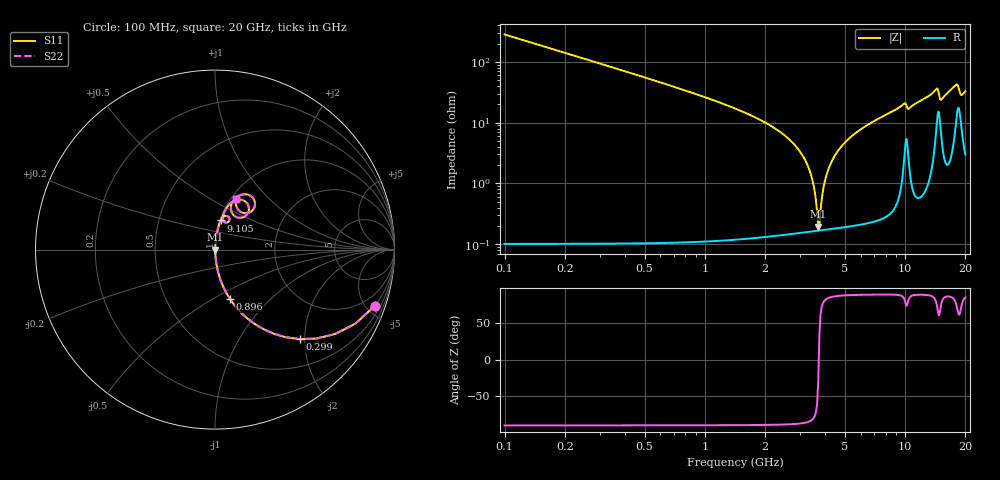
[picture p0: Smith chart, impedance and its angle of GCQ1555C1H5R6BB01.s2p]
!Murata Part Number: GCQ1555C1H5R6BB01
!These Parameters are Measured in Series Mode Connection
!Data Generated on Jan 08, 2026
!  o--ll--o
!Port1  Port2
!  o------o
!Operation Temp=25[degC], DC Bias Voltage=0[V]
!Freq. Start=100[MHz] Stop=20[GHz] 401[Steps]
# Hz S RI R 50
!Freq.(Hz) S11(Real) S11(Imag) S21(Real) S21(Imag) S12(Real) S12(Imag) S22(Real) S22(Imag)
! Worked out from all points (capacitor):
!   401 points, 100 MHz to 20 GHz, reference 50 ohm
!   read as one part in series: C = 5.6 pF near 199.5 MHz
!   lowest |Z| = 194 mohm at 3.682 GHz (marker M1)
!   series resonance near 3.706 GHz, so ESL is about 330 pH
!   S11 on the Smith chart (normalised r, x): 100 MHz: 1.00, -5.68; 299 MHz: 1.00, -1.89; 896 MHz: 1.00, -0.60; 9.105 GHz: 1.01, +0.34; 20 GHz: 1.06, +0.66
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1e8  0.8896 -0.3132  0.1104 0.3132  0.1104 0.3132  0.8896 -0.3132
2.99e8  0.4714 -0.4986  0.5286 0.4986  0.5286 0.4986  0.4714 -0.4986
5.4775e8  0.2053 -0.4029  0.7947 0.4029  0.7947 0.4029  0.2053 -0.4029
8.96e8  0.0827 -0.2736  0.9173 0.2736  0.9173 0.2736  0.0827 -0.2736
2.7865e9  0.00344 -0.0441  0.9966 0.0441  0.9966 0.0441  0.00344 -0.0441
3.43325e9  0.00175 -0.0117  0.9982 0.0117  0.9982 0.0117  0.00175 -0.0117
3.682e9  0.00166 -0.000988  0.9983 0.000988  0.9983 0.000988  0.00166 -0.000988
3.7815e9  0.00169 0.0031  0.9983 -0.0031  0.9983 -0.0031  0.00169 0.0031
3.93075e9  0.00179 0.00903  0.9982 -0.00903  0.9982 -0.00903  0.00179 0.00903
4.08e9  0.00195 0.0148  0.998 -0.0148  0.998 -0.0148  0.00195 0.0148
4.52775e9  0.00278 0.0309  0.9972 -0.0309  0.9972 -0.0309  0.00278 0.0309
5.3735e9  0.00539 0.0584  0.9946 -0.0584  0.9946 -0.0584  0.00539 0.0584
6.7665e9  0.0121 0.0984  0.9879 -0.0984  0.9879 -0.0984  0.0121 0.0984
9.10475e9  0.0319 0.1625  0.9681 -0.1625  0.9681 -0.1625  0.0319 0.1625
1.005e10  0.0786 0.178  0.9214 -0.178  0.9214 -0.178  0.0786 0.178
1.338325e10  0.0871 0.2593  0.9129 -0.2593  0.9129 -0.2593  0.0871 0.2593
1.437825e10  0.1702 0.2669  0.8298 -0.2669  0.8298 -0.2669  0.1702 0.2669
1.507475e10  0.1065 0.1892  0.8935 -0.1892  0.8935 -0.1892  0.1065 0.1892
1.67165e10  0.1169 0.2886  0.8831 -0.2886  0.8831 -0.2886  0.1169 0.2886
1.83085e10  0.223 0.2532  0.777 -0.2532  0.777 -0.2532  0.223 0.2532
1.895525e10  0.1468 0.2084  0.8532 -0.2084  0.8532 -0.2084  0.1468 0.2084
2e10  0.1183 0.2807  0.8817 -0.2807  0.8817 -0.2807  0.1183 0.2807
